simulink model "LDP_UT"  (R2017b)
settings: Solver=FixedStepDiscrete  StartTime=0.0  StopTime=10.0  FixedStep=0.01  RelTol=1e-3  EnableMultiTasking=on
undefined symbols (not defined in the file): ASWTYPE_FALSE, ASWTYPE_TRUE, CaCDP_ChrgTempNTCVoltTable_mV, CaCDP_ChrgTempTable_C, CaLDP_InletWtTempTable_C, CaLDP_InletWtVolt_mV, CaLDP_OutletWtTempTable_C, CaLDP_OutletWtVolt_mV, CcLDP_CC2SplyVolt_mV, CcLDP_CC2Uncon2ConTi_ms, CcLDP_CC2VoltThd_mV, CcLDP_DCChrgNegTempHiThrd_C, CcLDP_DCChrgNegTempMaxThrd_mV, CcLDP_DCChrgNegTempMinThrd_mV, CcLDP_DCChrgPosTempHiThrd_C, CcLDP_DCChrgPosTempMaxThrd_mV, CcLDP_DCChrgPosTempMinThrd_mV, CcLDP_DCSplyOnDebTi_ms, CcLDP_DCWakeVolt_V, CcLDP_IntWtTempHiThrd_C, CcLDP_IntWtTempMaxThrd_mV, CcLDP_IntWtTempMinThrd_mV, CcLDP_OutWtTempHiThrd_C, CcLDP_OutWtTempMaxThrd_mV, CcLDP_OutWtTempMinThrd_mV, Enum_CTCCtrCtlConnMode, Enum_LDPCC2St, Enum_LDPChrgGunState, Enum_ODPCCState, LDP_CONST2_NUMB, LDP_RUNTIME_MS
libraries: AIWAYS_Powertrain_BMS_lib x82
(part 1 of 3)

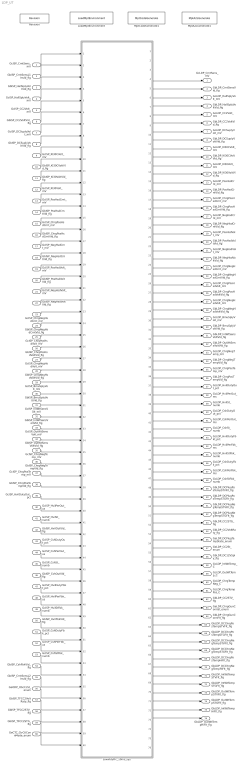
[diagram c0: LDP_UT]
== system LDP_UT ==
  GcISP_CrntSens_mV : Inport
  GbISP_CrntSensL1Invld_flg : Inport  Port=2
  GbISP_HallSplyVoltVld_flg : Inport  Port=3
  GcISP_HallSplyVolt_mV : Inport  Port=4
  GcISP_CC2Volt_mV : Inport  Port=5
  GbISP_CC2VoltVld_flg : Inport  Port=6
  GcISP_DCSuplyVolt_mV : Inport  Port=7
  GbISP_DCSuplyVoltVld_flg : Inport  Port=8
  GcISP_Kl30CVolt_mV : Inport  Port=9
  GbISP_Kl30CVoltVld_flg : Inport  Port=10
  GbISP_Kl30VoltVld_flg : Inport  Port=11
  GcISP_Kl30Volt_mV : Inport  Port=12
  GcISP_PosHsdCrnt_mV : Inport  Port=13
  GbISP_PosHsdCrntVld_flg : Inport  Port=14
  GcISP_ChrgPosHsdCrnt_mV : Inport  Port=15
  GbISP_ChrgPosHsdCrntVld_flg : Inport  Port=16
  GcISP_NegHsdCrnt_mV : Inport  Port=17
  GbISP_NegHsdCrntVld_flg : Inport  Port=18
  GcISP_PosHsdVolt_mV : Inport  Port=19
  GbISP_PosHsdVoltVld_flg : Inport  Port=20
  GcISP_NegHsdVolt_mV : Inport  Port=21
  GbISP_NegHsdVoltVld_flg : Inport  Port=22
  GcISP_ChrgNegHsdCrnt_mV : Inport  Port=23
  GbISP_ChrgNegHsdCrntVld_flg : Inport  Port=24
  GcISP_ChrgPosHsdVolt_mV : Inport  Port=25
  GbISP_ChrgPosHsdVoltVld_flg : Inport  Port=26
  GcISP_ChrgNegHsdVolt_mV : Inport  Port=27
  GbISP_ChrgNegHsdVoltVld_flg : Inport  Port=28
  GcISP_BmuSplyVolt_mV : Inport  Port=29
  GbISP_BmuSplyVoltVld_flg : Inport  Port=30
  GcISP_lntWtSensVolt_mV : Inport  Port=31
  GbISP_lntWtSensVoltVld_flg : Inport  Port=32
  GcISP_OutWtSensVolt_mV : Inport  Port=33
  GbISP_OutWtSensVoltVld_flg : Inport  Port=34
  GcISP_ChrgNegTemp_mV : Inport  Port=35
  GbISP_ChrgNegTempVld_flg : Inport  Port=36
  GcISP_ChrgPosTemp_mV : Inport  Port=37
  GbISP_ChrgPosTempVld_flg : Inport  Port=38
  GcISP_HvilDutyOut_pct : Inport  Port=39
  GcISP_HvilPerOut_us : Inport  Port=40
  GcISP_HvilSt_numb : Inport  Port=41
  GbISP_HvilOutVld_flg : Inport  Port=42
  GcISP_CshDutyOut_pct : Inport  Port=43
  GcISP_CshPerOut_us : Inport  Port=44
  GcISP_CshSt_numb : Inport  Port=45
  GbISP_CshOutVld_flg : Inport  Port=46
  GcISP_HvilDutyFbkt_pct : Inport  Port=47
  GcISP_HvilPerFbk_us : Inport  Port=48
  GcISP_HvilStFbk_numb : Inport  Port=49
  GbISP_HvilFbkVld_flg : Inport  Port=50
  GcISP_CshDutyFbk_pct : Inport  Port=51
  GcISP_CshPerFbk_us : Inport  Port=52
  GcISP_CshStFbk_numb : Inport  Port=53
  GbISP_CshFbkVld_flg : Inport  Port=54
  GbISP_CrntSensL2Invld_flg : Inport  Port=55
  GeODP_ObcCcSt_enum : Inport  Port=56
  GbISP_TFCC2VoltRaty_flg : Inport  Port=57
  GbISP_TFCC2STV_flg : Inport  Port=58
  GbISP_TFCC2STG_flg : Inport  Port=59
  GeCTC_CtrCtlConnMode_enum : Inport  Port=60
  LoadMptEnvironment : AIWAYS_Powertrain_BMS_lib/Config/LoadMptEnvironment  ProjectName=Comm  SuppierID=NewPlatformUAES
  LowVolyPrc_10ms_sys : Subsystem
  MptA2LGenerate1 : AIWAYS_Powertrain_BMS_lib/Config/MptA2LGenerate  SystemSampleTime=-1
  MptCodeGenerate1 : AIWAYS_Powertrain_BMS_lib/Config/MptCodeGenerate  SystemSampleTime=-1
  Revision : AIWAYS_Powertrain_BMS_lib/Config/Revision  curVersion='M104C110'  newVersion='M104C110'
  GcLDP_CrntSens_mV : Outport
  GbLDP_CrntSensVld_flg : Outport  Port=2
  GcLDP_HallSplyVolt_mV : Outport  Port=3
  GbLDP_HallSplyVoltVld_flg : Outport  Port=4
  GcLDP_CC2Volt_mV : Outport  Port=5
  GbLDP_CC2VoltVld_flg : Outport  Port=6
  GcLDP_DCSuplyVolt_mV : Outport  Port=7
  GbLDP_DCSuplyVoltVld_flg : Outport  Port=8
  GcLDP_Kl30CVolt_mV : Outport  Port=9
  GbLDP_Kl30CVoltVld_flg : Outport  Port=10
  GcLDP_Kl30Volt_mV : Outport  Port=11
  GbLDP_Kl30VoltVld_flg : Outport  Port=12
  GcLDP_PosHsdCrnt_mV : Outport  Port=13
  GbLDP_PosHsdCrntVld_flg : Outport  Port=14
  GcLDP_ChrgPosHsdCrnt_mV : Outport  Port=15
  GbLDP_ChrgPosHsdCrntVld_flg : Outport  Port=16
  GcLDP_NegHsdCrnt_mV : Outport  Port=17
  GbLDP_NegHsdCrntVld_flg : Outport  Port=18
  GcLDP_PosHsdVolt_mV : Outport  Port=19
  GbLDP_PosHsdVoltVld_flg : Outport  Port=20
  GcLDP_NegHsdVolt_mV : Outport  Port=21
  GbLDP_NegHsdVoltVld_flg : Outport  Port=22
  GcLDP_ChrgNegHsdCrnt_mV : Outport  Port=23
  GbLDP_ChrgNegHsdCrntVld_flg : Outport  Port=24
  GcLDP_ChrgPosHsdVolt_mV : Outport  Port=25
  GbLDP_ChrgPosHsdVoltVld_flg : Outport  Port=26
  GcLDP_ChrgNegHsdVolt_mV : Outport  Port=27
  GbLDP_ChrgNegHsdVoltVld_flg : Outport  Port=28
  GcLDP_BmuSplyVolt_mV : Outport  Port=29
  GbLDP_BmuSplyVoltVld_flg : Outport  Port=30
  GbLDP_lntWtSensVoltVld_flg : Outport  Port=31
  GbLDP_OutWtSensVoltVld_flg : Outport  Port=32
  GcLDP_ChrgNegTemp_mV : Outport  Port=33
  GbLDP_ChrgNegTempVld_flg : Outport  Port=34
  GcLDP_ChrgPosTemp_mV : Outport  Port=35
  GbLDP_ChrgPosTempVld_flg : Outport  Port=36
  GcLDP_HvilDutyOut_pct : Outport  Port=37
  GcLDP_HvilPerOut_ms : Outport  Port=38
  GcLDP_HvilSt_numb : Outport  Port=39
  GcLDP_CshDutyOut_pct : Outport  Port=40
  GcLDP_CshPerOut_ms : Outport  Port=41
  GcLDP_CshSt_numb : Outport  Port=42
  GcLDP_HvilDutyFbkt_pct : Outport  Port=43
  GcLDP_HvilPerFbk_ms : Outport  Port=44
  GcLDP_HvilStFbk_numb : Outport  Port=45
  GcLDP_CshDutyFbk_pct : Outport  Port=46
  GcLDP_CshPerFbk_ms : Outport  Port=47
  GcLDP_CshStFbk_numb : Outport  Port=48
  GbLDP_DCPlugPosTempSTVFlt_flg : Outport  Port=49
  GbLDP_DCPlugPosTempSTGFlt_flg : Outport  Port=50
  GbLDP_DCPlugNegTempSTVFlt_flg : Outport  Port=51
  GbLDP_DCPlugNegTempSTGFlt_flg : Outport  Port=52
  GbLDP_CC2STG_flg : Outport  Port=53
  GbLDP_CC2VoltRaty_flg : Outport  Port=54
  GeLDP_DCPlugTempState_enum : Outport  Port=55
  GbLDP_DC12VSply_flg : Outport  Port=56
  GeLDP_CC2St_enum : Outport  Port=57
  GcLDP_lntWtTemp_C : Outport  Port=58
  GcLDP_OutWtTemp_C : Outport  Port=59
  GcLDP_ChrgTempNeg_C : Outport  Port=60
  GcLDP_ChrgTempPos_C : Outport  Port=61
  GbLDP_CC2STV_flg : Outport  Port=62
  GeLDP_ChrgGunConnSt_enum : Outport  Port=63
  GbLDP_ChrgGunConnFlt_flg : Outport  Port=64
  GbLDP_DCChrgPosTempSTVFlt_flg : Outport  Port=65
  GbLDP_DCChrgPosTempSTGFlt_flg : Outport  Port=66
  GbLDP_DCChrgNegTempSTVFlt_flg : Outport  Port=67
  GbLDP_DCChrgNegTempSTGFlt_flg : Outport  Port=68
  GbLDP_DCChrgPosTempHiFlt_flg : Outport  Port=69
  GbLDP_DCChrgNegTempHiFlt_flg : Outport  Port=70
  GbLDP_IntWtTempSTVFlt_flg : Outport  Port=71
  GbLDP_IntWtTempSTGFlt_flg : Outport  Port=72
  GbLDP_OutWtTempSTVFlt_flg : Outport  Port=73
  GbLDP_OutWtTempSTGFlt_flg : Outport  Port=74
  GbLDP_IntWtTempHiFlt_flg : Outport  Port=75
  GbLDP_OutWtTempHiFlt_flg : Outport  Port=76
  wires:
  GbISP_DCSuplyVoltVld_flg/1 -> LowVolyPrc_10ms_sys/8(GbISP_DCSuplyVoltVld_flg)
  GbISP_CC2VoltVld_flg/1 -> LowVolyPrc_10ms_sys/6(GbISP_CC2VoltVld_flg)
  LowVolyPrc_10ms_sys/47(GcLDP_CshPerFbk_ms) -> GcLDP_CshPerFbk_ms/1
  LowVolyPrc_10ms_sys/66(GbLDP_DCChrgPosTempSTGFlt_flg) -> GbLDP_DCChrgPosTempSTGFlt_flg/1
  LowVolyPrc_10ms_sys/19(GcLDP_PosHsdVolt_mV) -> GcLDP_PosHsdVolt_mV/1
  GbISP_TFCC2VoltRaty_flg/1 -> LowVolyPrc_10ms_sys/57(GbISP_TFCC2VoltRaty_flg)
  GbISP_PosHsdVoltVld_flg/1 -> LowVolyPrc_10ms_sys/20(GbISP_PosHsdVoltVld_flg)
  LowVolyPrc_10ms_sys/1(GcLDP_CrntSens_mV) -> GcLDP_CrntSens_mV/1
  GcISP_ChrgNegHsdCrnt_mV/1 -> LowVolyPrc_10ms_sys/23(GcISP_ChrgNegHsdCrnt_mV)
  LowVolyPrc_10ms_sys/44(GcLDP_HvilPerFbk_ms) -> GcLDP_HvilPerFbk_ms/1
  LowVolyPrc_10ms_sys/12(GbLDP_Kl30VoltVld_flg) -> GbLDP_Kl30VoltVld_flg/1
  LowVolyPrc_10ms_sys/3(GcLDP_HallSplyVolt_mV) -> GcLDP_HallSplyVolt_mV/1
  LowVolyPrc_10ms_sys/5(GcLDP_CC2Volt_mV) -> GcLDP_CC2Volt_mV/1
  GeCTC_CtrCtlConnMode_enum/1 -> LowVolyPrc_10ms_sys/60(GeCTC_CtrCtlConnMode_enum)
  GcISP_NegHsdVolt_mV/1 -> LowVolyPrc_10ms_sys/21(GcISP_NegHsdVolt_mV)
  LowVolyPrc_10ms_sys/56(GeLDP_CC2St_enum) -> GeLDP_CC2St_enum/1
  GbISP_NegHsdVoltVld_flg/1 -> LowVolyPrc_10ms_sys/22(GbISP_NegHsdVoltVld_flg)
  GcISP_BmuSplyVolt_mV/1 -> LowVolyPrc_10ms_sys/29(GcISP_BmuSplyVolt_mV)
  LowVolyPrc_10ms_sys/36(GbLDP_ChrgPosTempVld_flg) -> GbLDP_ChrgPosTempVld_flg/1
  LowVolyPrc_10ms_sys/24(GbLDP_ChrgNegHsdCrntVld_flg) -> GbLDP_ChrgNegHsdCrntVld_flg/1
  GcISP_NegHsdCrnt_mV/1 -> LowVolyPrc_10ms_sys/17(GcISP_NegHsdCrnt_mV)
  GbISP_TFCC2STG_flg/1 -> LowVolyPrc_10ms_sys/59(GbISP_TFCC2STG_flg)
  LowVolyPrc_10ms_sys/15(GcLDP_ChrgPosHsdCrnt_mV) -> GcLDP_ChrgPosHsdCrnt_mV/1
  LowVolyPrc_10ms_sys/51(GbLDP_DCPlugNegTempSTVFlt_flg) -> GbLDP_DCPlugNegTempSTVFlt_flg/1
  LowVolyPrc_10ms_sys/45(GcLDP_HvilStFbk_numb) -> GcLDP_HvilStFbk_numb/1
  LowVolyPrc_10ms_sys/11(GcLDP_Kl30Volt_mV) -> GcLDP_Kl30Volt_mV/1
  LowVolyPrc_10ms_sys/37(GcLDP_HvilDutyOut_pct) -> GcLDP_HvilDutyOut_pct/1
  GbISP_BmuSplyVoltVld_flg/1 -> LowVolyPrc_10ms_sys/30(GbISP_BmuSplyVoltVld_flg)
  LowVolyPrc_10ms_sys/65(GbLDP_DCChrgPosTempSTVFlt_flg) -> GbLDP_DCChrgPosTempSTVFlt_flg/1
  GbISP_HallSplyVoltVld_flg/1 -> LowVolyPrc_10ms_sys/3(GbISP_HallSplyVoltVld_flg)
  LowVolyPrc_10ms_sys/63(GeLDP_ChrgGunConnSt_enum) -> GeLDP_ChrgGunConnSt_enum/1
  GeODP_ObcCcSt_enum/1 -> LowVolyPrc_10ms_sys/56(GeODP_ObcCcSt_enum)
  GbISP_CshOutVld_flg/1 -> LowVolyPrc_10ms_sys/46(GbISP_CshOutVld_flg)
  LowVolyPrc_10ms_sys/34(GbLDP_ChrgNegTempVld_flg) -> GbLDP_ChrgNegTempVld_flg/1
  GbISP_CrntSensL1Invld_flg/1 -> LowVolyPrc_10ms_sys/2(GbISP_CrntSensL1Invld_flg)
  LowVolyPrc_10ms_sys/25(GcLDP_ChrgPosHsdVolt_mV) -> GcLDP_ChrgPosHsdVolt_mV/1
  LowVolyPrc_10ms_sys/22(GbLDP_NegHsdVoltVld_flg) -> GbLDP_NegHsdVoltVld_flg/1
  LowVolyPrc_10ms_sys/16(GbLDP_ChrgPosHsdCrntVld_flg) -> GbLDP_ChrgPosHsdCrntVld_flg/1
  GcISP_PosHsdCrnt_mV/1 -> LowVolyPrc_10ms_sys/13(GcISP_PosHsdCrnt_mV)
  LowVolyPrc_10ms_sys/20(GbLDP_PosHsdVoltVld_flg) -> GbLDP_PosHsdVoltVld_flg/1
  GcISP_DCSuplyVolt_mV/1 -> LowVolyPrc_10ms_sys/7(GcISP_DCSuplyVolt_mV)
  LowVolyPrc_10ms_sys/18(GbLDP_NegHsdCrntVld_flg) -> GbLDP_NegHsdCrntVld_flg/1
  LowVolyPrc_10ms_sys/14(GbLDP_PosHsdCrntVld_flg) -> GbLDP_PosHsdCrntVld_flg/1
  LowVolyPrc_10ms_sys/21(GcLDP_NegHsdVolt_mV) -> GcLDP_NegHsdVolt_mV/1
  GbISP_PosHsdCrntVld_flg/1 -> LowVolyPrc_10ms_sys/14(GbISP_PosHsdCrntVld_flg)
  LowVolyPrc_10ms_sys/13(GcLDP_PosHsdCrnt_mV) -> GcLDP_PosHsdCrnt_mV/1
  LowVolyPrc_10ms_sys/30(GbLDP_BmuSplyVoltVld_flg) -> GbLDP_BmuSplyVoltVld_flg/1
  LowVolyPrc_10ms_sys/8(GbLDP_DCSuplyVoltVld_flg) -> GbLDP_DCSuplyVoltVld_flg/1
  LowVolyPrc_10ms_sys/54(GbLDP_CC2VoltRaty_flg) -> GbLDP_CC2VoltRaty_flg/1
  LowVolyPrc_10ms_sys/9(GcLDP_Kl30CVolt_mV) -> GcLDP_Kl30CVolt_mV/1
  LowVolyPrc_10ms_sys/26(GbLDP_ChrgPosHsdVoltVld_flg) -> GbLDP_ChrgPosHsdVoltVld_flg/1
  GcISP_Kl30Volt_mV/1 -> LowVolyPrc_10ms_sys/12(GcISP_Kl30Volt_mV)
  GbISP_Kl30VoltVld_flg/1 -> LowVolyPrc_10ms_sys/11(GbISP_Kl30VoltVld_flg)
  GbISP_Kl30CVoltVld_flg/1 -> LowVolyPrc_10ms_sys/10(GbISP_Kl30CVoltVld_flg)
  LowVolyPrc_10ms_sys/17(GcLDP_NegHsdCrnt_mV) -> GcLDP_NegHsdCrnt_mV/1
  GcISP_Kl30CVolt_mV/1 -> LowVolyPrc_10ms_sys/9(GcISP_Kl30CVolt_mV)
  LowVolyPrc_10ms_sys/31(GbLDP_lntWtSensVoltVld_flg) -> GbLDP_lntWtSensVoltVld_flg/1
  LowVolyPrc_10ms_sys/43(GcLDP_HvilDutyFbkt_pct) -> GcLDP_HvilDutyFbkt_pct/1
  LowVolyPrc_10ms_sys/7(GcLDP_DCSuplyVolt_mV) -> GcLDP_DCSuplyVolt_mV/1
  LowVolyPrc_10ms_sys/35(GcLDP_ChrgPosTemp_mV) -> GcLDP_ChrgPosTemp_mV/1
  LowVolyPrc_10ms_sys/32(GbLDP_OutWtSensVoltVld_flg) -> GbLDP_OutWtSensVoltVld_flg/1
  GbISP_ChrgPosHsdCrntVld_flg/1 -> LowVolyPrc_10ms_sys/16(GbISP_ChrgPosHsdCrntVld_flg)
  LowVolyPrc_10ms_sys/28(GbLDP_ChrgNegHsdVoltVld_flg) -> GbLDP_ChrgNegHsdVoltVld_flg/1
  GbISP_ChrgNegHsdCrntVld_flg/1 -> LowVolyPrc_10ms_sys/24(GbISP_ChrgNegHsdCrntVld_flg)
  GcISP_PosHsdVolt_mV/1 -> LowVolyPrc_10ms_sys/19(GcISP_PosHsdVolt_mV)
  LowVolyPrc_10ms_sys/10(GbLDP_Kl30CVoltVld_flg) -> GbLDP_Kl30CVoltVld_flg/1
  GcISP_CshPerFbk_us/1 -> LowVolyPrc_10ms_sys/52(GcISP_CshPerFbk_us)
  GbISP_HvilFbkVld_flg/1 -> LowVolyPrc_10ms_sys/50(GbISP_HvilFbkVld_flg)
  LowVolyPrc_10ms_sys/70(GbLDP_DCChrgNegTempHiFlt_flg) -> GbLDP_DCChrgNegTempHiFlt_flg/1
  GcISP_HvilPerOut_us/1 -> LowVolyPrc_10ms_sys/40(GcISP_HvilPerOut_us)
  GcISP_CshDutyOut_pct/1 -> LowVolyPrc_10ms_sys/43(GcISP_CshDutyOut_pct)
  LowVolyPrc_10ms_sys/49(GbLDP_DCPlugPosTempSTVFlt_flg) -> GbLDP_DCPlugPosTempSTVFlt_flg/1
  LowVolyPrc_10ms_sys/57(GbLDP_DC12VSply_flg) -> GbLDP_DC12VSply_flg/1
  GcISP_OutWtSensVolt_mV/1 -> LowVolyPrc_10ms_sys/33(GcISP_OutWtSensVolt_mV)
  LowVolyPrc_10ms_sys/40(GcLDP_CshDutyOut_pct) -> GcLDP_CshDutyOut_pct/1
  GbISP_ChrgNegTempVld_flg/1 -> LowVolyPrc_10ms_sys/36(GbISP_ChrgNegTempVld_flg)
  GcISP_ChrgPosHsdCrnt_mV/1 -> LowVolyPrc_10ms_sys/15(GcISP_ChrgPosHsdCrnt_mV)
  LowVolyPrc_10ms_sys/61(GcLDP_ChrgTempPos_C) -> GcLDP_ChrgTempPos_C/1
  GcISP_HvilDutyFbkt_pct/1 -> LowVolyPrc_10ms_sys/47(GcISP_HvilDutyFbkt_pct)
  LowVolyPrc_10ms_sys/52(GbLDP_DCPlugNegTempSTGFlt_flg) -> GbLDP_DCPlugNegTempSTGFlt_flg/1
  GcISP_ChrgPosTemp_mV/1 -> LowVolyPrc_10ms_sys/37(GcISP_ChrgPosTemp_mV)
  LowVolyPrc_10ms_sys/60(GcLDP_ChrgTempNeg_C) -> GcLDP_ChrgTempNeg_C/1
  LowVolyPrc_10ms_sys/41(GcLDP_CshPerOut_ms) -> GcLDP_CshPerOut_ms/1
  GbISP_CrntSensL2Invld_flg/1 -> LowVolyPrc_10ms_sys/55(GbISP_CrntSensL2Invld_flg)
  LowVolyPrc_10ms_sys/48(GcLDP_CshStFbk_numb) -> GcLDP_CshStFbk_numb/1
  LowVolyPrc_10ms_sys/2(GbLDP_CrntSensVld_flg) -> GbLDP_CrntSensVld_flg/1
  LowVolyPrc_10ms_sys/74(GbLDP_OutWtTempSTGFlt_flg) -> GbLDP_OutWtTempSTGFlt_flg/1
  GcISP_ChrgNegTemp_mV/1 -> LowVolyPrc_10ms_sys/35(GcISP_ChrgNegTemp_mV)
  LowVolyPrc_10ms_sys/59(GcLDP_OutWtTemp_C) -> GcLDP_OutWtTemp_C/1
  LowVolyPrc_10ms_sys/42(GcLDP_CshSt_numb) -> GcLDP_CshSt_numb/1
  LowVolyPrc_10ms_sys/76(GbLDP_OutWtTempHiFlt_flg) -> GbLDP_OutWtTempHiFlt_flg/1
  GcISP_ChrgNegHsdVolt_mV/1 -> LowVolyPrc_10ms_sys/27(GcISP_ChrgNegHsdVolt_mV)
  GcISP_HallSplyVolt_mV/1 -> LowVolyPrc_10ms_sys/4(GcISP_HallSplyVolt_mV)
  LowVolyPrc_10ms_sys/71(GbLDP_IntWtTempSTVFlt_flg) -> GbLDP_IntWtTempSTVFlt_flg/1
  LowVolyPrc_10ms_sys/75(GbLDP_IntWtTempHiFlt_flg) -> GbLDP_IntWtTempHiFlt_flg/1
  GbISP_OutWtSensVoltVld_flg/1 -> LowVolyPrc_10ms_sys/34(GbISP_OutWtSensVoltVld_flg)
  GcISP_HvilStFbk_numb/1 -> LowVolyPrc_10ms_sys/49(GcISP_HvilStFbk_numb)
  LowVolyPrc_10ms_sys/67(GbLDP_DCChrgNegTempSTVFlt_flg) -> GbLDP_DCChrgNegTempSTVFlt_flg/1
  GbISP_ChrgPosHsdVoltVld_flg/1 -> LowVolyPrc_10ms_sys/26(GbISP_ChrgPosHsdVoltVld_flg)
  LowVolyPrc_10ms_sys/33(GcLDP_ChrgNegTemp_mV) -> GcLDP_ChrgNegTemp_mV/1
  GbISP_TFCC2STV_flg/1 -> LowVolyPrc_10ms_sys/58(GbISP_TFCC2STV_flg)
  GcISP_CshSt_numb/1 -> LowVolyPrc_10ms_sys/45(GcISP_CshSt_numb)
  GcISP_HvilPerFbk_us/1 -> LowVolyPrc_10ms_sys/48(GcISP_HvilPerFbk_us)
  LowVolyPrc_10ms_sys/53(GbLDP_CC2STG_flg) -> GbLDP_CC2STG_flg/1
  GbISP_lntWtSensVoltVld_flg/1 -> LowVolyPrc_10ms_sys/32(GbISP_lntWtSensVoltVld_flg)
  LowVolyPrc_10ms_sys/73(GbLDP_OutWtTempSTVFlt_flg) -> GbLDP_OutWtTempSTVFlt_flg/1
  LowVolyPrc_10ms_sys/39(GcLDP_HvilSt_numb) -> GcLDP_HvilSt_numb/1
  LowVolyPrc_10ms_sys/64(GbLDP_ChrgGunConnFlt_flg) -> GbLDP_ChrgGunConnFlt_flg/1
  GbISP_NegHsdCrntVld_flg/1 -> LowVolyPrc_10ms_sys/18(GbISP_NegHsdCrntVld_flg)
  GcISP_HvilSt_numb/1 -> LowVolyPrc_10ms_sys/41(GcISP_HvilSt_numb)
  GcISP_ChrgPosHsdVolt_mV/1 -> LowVolyPrc_10ms_sys/25(GcISP_ChrgPosHsdVolt_mV)
  GcISP_CshDutyFbk_pct/1 -> LowVolyPrc_10ms_sys/51(GcISP_CshDutyFbk_pct)
  LowVolyPrc_10ms_sys/55(GeLDP_DCPlugTempState_enum) -> GeLDP_DCPlugTempState_enum/1
  LowVolyPrc_10ms_sys/38(GcLDP_HvilPerOut_ms) -> GcLDP_HvilPerOut_ms/1
  GcISP_lntWtSensVolt_mV/1 -> LowVolyPrc_10ms_sys/31(GcISP_lntWtSensVolt_mV)
  GbISP_HvilOutVld_flg/1 -> LowVolyPrc_10ms_sys/42(GbISP_HvilOutVld_flg)
  LowVolyPrc_10ms_sys/72(GbLDP_IntWtTempSTGFlt_flg) -> GbLDP_IntWtTempSTGFlt_flg/1
  GbISP_CshFbkVld_flg/1 -> LowVolyPrc_10ms_sys/54(GbISP_CshFbkVld_flg)
  GcISP_CC2Volt_mV/1 -> LowVolyPrc_10ms_sys/5(GcISP_CC2Volt_mV)
  LowVolyPrc_10ms_sys/58(GcLDP_lntWtTemp_C) -> GcLDP_lntWtTemp_C/1
  LowVolyPrc_10ms_sys/29(GcLDP_BmuSplyVolt_mV) -> GcLDP_BmuSplyVolt_mV/1
  LowVolyPrc_10ms_sys/6(GbLDP_CC2VoltVld_flg) -> GbLDP_CC2VoltVld_flg/1
  LowVolyPrc_10ms_sys/50(GbLDP_DCPlugPosTempSTGFlt_flg) -> GbLDP_DCPlugPosTempSTGFlt_flg/1
  GcISP_CshPerOut_us/1 -> LowVolyPrc_10ms_sys/44(GcISP_CshPerOut_us)
  LowVolyPrc_10ms_sys/4(GbLDP_HallSplyVoltVld_flg) -> GbLDP_HallSplyVoltVld_flg/1
  LowVolyPrc_10ms_sys/27(GcLDP_ChrgNegHsdVolt_mV) -> GcLDP_ChrgNegHsdVolt_mV/1
  GcISP_CshStFbk_numb/1 -> LowVolyPrc_10ms_sys/53(GcISP_CshStFbk_numb)
  LowVolyPrc_10ms_sys/68(GbLDP_DCChrgNegTempSTGFlt_flg) -> GbLDP_DCChrgNegTempSTGFlt_flg/1
  GbISP_ChrgPosTempVld_flg/1 -> LowVolyPrc_10ms_sys/38(GbISP_ChrgPosTempVld_flg)
  GcISP_CrntSens_mV/1 -> LowVolyPrc_10ms_sys/1(GcISP_CrntSens_mV)
  LowVolyPrc_10ms_sys/69(GbLDP_DCChrgPosTempHiFlt_flg) -> GbLDP_DCChrgPosTempHiFlt_flg/1
  GbISP_ChrgNegHsdVoltVld_flg/1 -> LowVolyPrc_10ms_sys/28(GbISP_ChrgNegHsdVoltVld_flg)
  GcISP_HvilDutyOut_pct/1 -> LowVolyPrc_10ms_sys/39(GcISP_HvilDutyOut_pct)
  LowVolyPrc_10ms_sys/46(GcLDP_CshDutyFbk_pct) -> GcLDP_CshDutyFbk_pct/1
  LowVolyPrc_10ms_sys/62(GbLDP_CC2STV_flg) -> GbLDP_CC2STV_flg/1
  LowVolyPrc_10ms_sys/23(GcLDP_ChrgNegHsdCrnt_mV) -> GcLDP_ChrgNegHsdCrnt_mV/1

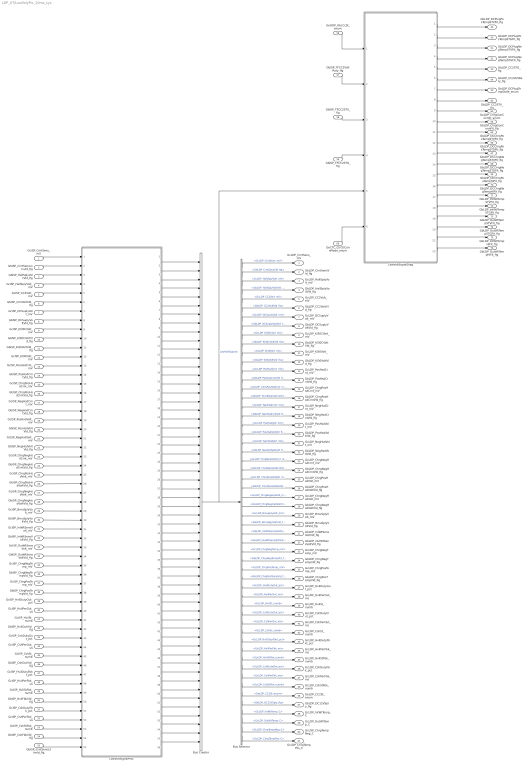
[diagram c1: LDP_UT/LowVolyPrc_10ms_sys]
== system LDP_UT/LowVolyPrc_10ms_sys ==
  GcISP_CrntSens_mV : Inport
  GbISP_CrntSensL1Invld_flg : Inport  Port=2
  GbISP_HallSplyVoltVld_flg : Inport  Port=3
  GcISP_HallSplyVolt_mV : Inport  Port=4
  GcISP_CC2Volt_mV : Inport  Port=5
  GbISP_CC2VoltVld_flg : Inport  Port=6
  GcISP_DCSuplyVolt_mV : Inport  Port=7
  GbISP_DCSuplyVoltVld_flg : Inport  Port=8
  GcISP_Kl30CVolt_mV : Inport  Port=9
  GbISP_Kl30CVoltVld_flg : Inport  Port=10
  GbISP_Kl30VoltVld_flg : Inport  Port=11
  GcISP_Kl30Volt_mV : Inport  Port=12
  GcISP_PosHsdCrnt_mV : Inport  Port=13
  GbISP_PosHsdCrntVld_flg : Inport  Port=14
  GcISP_ChrgPosHsdCrnt_mV : Inport  Port=15
  GbISP_ChrgPosHsdCrntVld_flg : Inport  Port=16
  GcISP_NegHsdCrnt_mV : Inport  Port=17
  GbISP_NegHsdCrntVld_flg : Inport  Port=18
  GcISP_PosHsdVolt_mV : Inport  Port=19
  GbISP_PosHsdVoltVld_flg : Inport  Port=20
  GcISP_NegHsdVolt_mV : Inport  Port=21
  GbISP_NegHsdVoltVld_flg : Inport  Port=22
  GcISP_ChrgNegHsdCrnt_mV : Inport  Port=23
  GbISP_ChrgNegHsdCrntVld_flg : Inport  Port=24
  GcISP_ChrgPosHsdVolt_mV : Inport  Port=25
  GbISP_ChrgPosHsdVoltVld_flg : Inport  Port=26
  GcISP_ChrgNegHsdVolt_mV : Inport  Port=27
  GbISP_ChrgNegHsdVoltVld_flg : Inport  Port=28
  GcISP_BmuSplyVolt_mV : Inport  Port=29
  GbISP_BmuSplyVoltVld_flg : Inport  Port=30
  GcISP_lntWtSensVolt_mV : Inport  Port=31
  GbISP_lntWtSensVoltVld_flg : Inport  Port=32
  GcISP_OutWtSensVolt_mV : Inport  Port=33
  GbISP_OutWtSensVoltVld_flg : Inport  Port=34
  GcISP_ChrgNegTemp_mV : Inport  Port=35
  GbISP_ChrgNegTempVld_flg : Inport  Port=36
  GcISP_ChrgPosTemp_mV : Inport  Port=37
  GbISP_ChrgPosTempVld_flg : Inport  Port=38
  GcISP_HvilDutyOut_pct : Inport  Port=39
  GcISP_HvilPerOut_us : Inport  Port=40
  GcISP_HvilSt_numb : Inport  Port=41
  GbISP_HvilOutVld_flg : Inport  Port=42
  GcISP_CshDutyOut_pct : Inport  Port=43
  GcISP_CshPerOut_us : Inport  Port=44
  GcISP_CshSt_numb : Inport  Port=45
  GbISP_CshOutVld_flg : Inport  Port=46
  GcISP_HvilDutyFbkt_pct : Inport  Port=47
  GcISP_HvilPerFbk_us : Inport  Port=48
  GcISP_HvilStFbk_numb : Inport  Port=49
  GbISP_HvilFbkVld_flg : Inport  Port=50
  GcISP_CshDutyFbk_pct : Inport  Port=51
  GcISP_CshPerFbk_us : Inport  Port=52
  GcISP_CshStFbk_numb : Inport  Port=53
  GbISP_CshFbkVld_flg : Inport  Port=54
  GbISP_CrntSensL2Invld_flg : Inport  Port=55
  GeODP_ObcCcSt_enum : Inport  Port=56
  GbISP_TFCC2VoltRaty_flg : Inport  Port=57
  GbISP_TFCC2STV_flg : Inport  Port=58
  GbISP_TFCC2STG_flg : Inport  Port=59
  GeCTC_CtrCtlConnMode_enum : Inport  Port=60
  Bus Creator : BusCreator  Inputs=56
  Bus Selector : BusSelector  OutputSignals=GcLDP_CrntSens_mV,GbLDP_CrntSensVld_flg,GcLDP_HallSplyVolt_mV,GbLDP_HallSplyVoltVld_flg,GcLDP_CC2Volt_mV,GbLDP_CC2VoltVld_flg,GcLDP_DCSuplyVolt_mV,GbLDP_DCSuplyVoltVld_flg,GcLDP_Kl30CVolt_mV,GbLDP_Kl30CVoltVld_flg,GcLDP_Kl30Volt_mV,GbLDP_Kl30VoltVld_flg,GcLDP_PosHsdCrnt_mV,GbLDP_PosHsdCrntVld_flg,GcLDP_ChrgPosHsdCrnt_mV,GbLDP_ChrgPosHsdCrntVld_flg,GcLDP_NegHsdCrnt_mV,GbLDP_NegHsdCrntVld_flg,GcLDP_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
  LowVoltSignalDiag : Subsystem
  LowVoltSignalProc : Subsystem
  GcLDP_CrntSens_mV : Outport
  GbLDP_CrntSensVld_flg : Outport  Port=2
  GcLDP_HallSplyVolt_mV : Outport  Port=3
  GbLDP_HallSplyVoltVld_flg : Outport  Port=4
  GcLDP_CC2Volt_mV : Outport  Port=5
  GbLDP_CC2VoltVld_flg : Outport  Port=6
  GcLDP_DCSuplyVolt_mV : Outport  Port=7
  GbLDP_DCSuplyVoltVld_flg : Outport  Port=8
  GcLDP_Kl30CVolt_mV : Outport  Port=9
  GbLDP_Kl30CVoltVld_flg : Outport  Port=10
  GcLDP_Kl30Volt_mV : Outport  Port=11
  GbLDP_Kl30VoltVld_flg : Outport  Port=12
  GcLDP_PosHsdCrnt_mV : Outport  Port=13
  GbLDP_PosHsdCrntVld_flg : Outport  Port=14
  GcLDP_ChrgPosHsdCrnt_mV : Outport  Port=15
  GbLDP_ChrgPosHsdCrntVld_flg : Outport  Port=16
  GcLDP_NegHsdCrnt_mV : Outport  Port=17
  GbLDP_NegHsdCrntVld_flg : Outport  Port=18
  GcLDP_PosHsdVolt_mV : Outport  Port=19
  GbLDP_PosHsdVoltVld_flg : Outport  Port=20
  GcLDP_NegHsdVolt_mV : Outport  Port=21
  GbLDP_NegHsdVoltVld_flg : Outport  Port=22
  GcLDP_ChrgNegHsdCrnt_mV : Outport  Port=23
  GbLDP_ChrgNegHsdCrntVld_flg : Outport  Port=24
  GcLDP_ChrgPosHsdVolt_mV : Outport  Port=25
  GbLDP_ChrgPosHsdVoltVld_flg : Outport  Port=26
  GcLDP_ChrgNegHsdVolt_mV : Outport  Port=27
  GbLDP_ChrgNegHsdVoltVld_flg : Outport  Port=28
  GcLDP_BmuSplyVolt_mV : Outport  Port=29
  GbLDP_BmuSplyVoltVld_flg : Outport  Port=30
  GbLDP_lntWtSensVoltVld_flg : Outport  Port=31
  GbLDP_OutWtSensVoltVld_flg : Outport  Port=32
  GcLDP_ChrgNegTemp_mV : Outport  Port=33
  GbLDP_ChrgNegTempVld_flg : Outport  Port=34
  GcLDP_ChrgPosTemp_mV : Outport  Port=35
  GbLDP_ChrgPosTempVld_flg : Outport  Port=36
  GcLDP_HvilDutyOut_pct : Outport  Port=37
  GcLDP_HvilPerOut_ms : Outport  Port=38
  GcLDP_HvilSt_numb : Outport  Port=39
  GcLDP_CshDutyOut_pct : Outport  Port=40
  GcLDP_CshPerOut_ms : Outport  Port=41
  GcLDP_CshSt_numb : Outport  Port=42
  GcLDP_HvilDutyFbkt_pct : Outport  Port=43
  GcLDP_HvilPerFbk_ms : Outport  Port=44
  GcLDP_HvilStFbk_numb : Outport  Port=45
  GcLDP_CshDutyFbk_pct : Outport  Port=46
  GcLDP_CshPerFbk_ms : Outport  Port=47
  GcLDP_CshStFbk_numb : Outport  Port=48
  GbLDP_DCPlugPosTempSTVFlt_flg : Outport  Port=49
  GbLDP_DCPlugPosTempSTGFlt_flg : Outport  Port=50
  GbLDP_DCPlugNegTempSTVFlt_flg : Outport  Port=51
  GbLDP_DCPlugNegTempSTGFlt_flg : Outport  Port=52
  GbLDP_CC2STG_flg : Outport  Port=53
  GbLDP_CC2VoltRaty_flg : Outport  Port=54
  GeLDP_DCPlugTempState_enum : Outport  Port=55
  GeLDP_CC2St_enum : Outport  Port=56
  GbLDP_DC12VSply_flg : Outport  Port=57
  GcLDP_lntWtTemp_C : Outport  Port=58
  GcLDP_OutWtTemp_C : Outport  Port=59
  GcLDP_ChrgTempNeg_C : Outport  Port=60
  GcLDP_ChrgTempPos_C : Outport  Port=61
  GbLDP_CC2STV_flg : Outport  Port=62
  GeLDP_ChrgGunConnSt_enum : Outport  Port=63
  GbLDP_ChrgGunConnFlt_flg : Outport  Port=64
  GbLDP_DCChrgPosTempSTVFlt_flg : Outport  Port=65
  GbLDP_DCChrgPosTempSTGFlt_flg : Outport  Port=66
  GbLDP_DCChrgNegTempSTVFlt_flg : Outport  Port=67
  GbLDP_DCChrgNegTempSTGFlt_flg : Outport  Port=68
  GbLDP_DCChrgPosTempHiFlt_flg : Outport  Port=69
  GbLDP_DCChrgNegTempHiFlt_flg : Outport  Port=70
  GbLDP_IntWtTempSTVFlt_flg : Outport  Port=71
  GbLDP_IntWtTempSTGFlt_flg : Outport  Port=72
  GbLDP_OutWtTempSTVFlt_flg : Outport  Port=73
  GbLDP_OutWtTempSTGFlt_flg : Outport  Port=74
  GbLDP_IntWtTempHiFlt_flg : Outport  Port=75
  GbLDP_OutWtTempHiFlt_flg : Outport  Port=76
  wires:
  GcISP_CrntSens_mV/1 -> LowVoltSignalProc/1(GcISP_CrntSens_mV)
  GbISP_CrntSensL1Invld_flg/1 -> LowVoltSignalProc/2(GbISP_CrntSensL1Invld_flg)
  GbISP_HallSplyVoltVld_flg/1 -> LowVoltSignalProc/3(GbISP_HallSplyVoltVld_flg)
  GcISP_HallSplyVolt_mV/1 -> LowVoltSignalProc/4(GcISP_HallSplyVolt_mV)
  GcISP_CC2Volt_mV/1 -> LowVoltSignalProc/5(GcISP_CC2Volt_mV)
  GbISP_CC2VoltVld_flg/1 -> LowVoltSignalProc/6(GbISP_CC2VoltVld_flg)
  GcISP_DCSuplyVolt_mV/1 -> LowVoltSignalProc/7(GcISP_DCSuplyVolt_mV)
  GbISP_DCSuplyVoltVld_flg/1 -> LowVoltSignalProc/8(GbISP_DCSuplyVoltVld_flg)
  GbISP_Kl30VoltVld_flg/1 -> LowVoltSignalProc/11(GbISP_Kl30VoltVld_flg)
  GcISP_Kl30Volt_mV/1 -> LowVoltSignalProc/12(GcISP_Kl30Volt_mV)
  GcISP_PosHsdCrnt_mV/1 -> LowVoltSignalProc/13(GcISP_PosHsdCrnt_mV)
  GbISP_PosHsdCrntVld_flg/1 -> LowVoltSignalProc/14(GbISP_PosHsdCrntVld_flg)
  GcISP_ChrgPosHsdCrnt_mV/1 -> LowVoltSignalProc/15(GcISP_ChrgPosHsdCrnt_mV)
  GbISP_ChrgPosHsdCrntVld_flg/1 -> LowVoltSignalProc/16(GbISP_ChrgPosHsdCrntVld_flg)
  GcISP_NegHsdCrnt_mV/1 -> LowVoltSignalProc/17(GcISP_NegHsdCrnt_mV)
  GbISP_NegHsdCrntVld_flg/1 -> LowVoltSignalProc/18(GbISP_NegHsdCrntVld_flg)
  GcISP_PosHsdVolt_mV/1 -> LowVoltSignalProc/19(GcISP_PosHsdVolt_mV)
  GbISP_PosHsdVoltVld_flg/1 -> LowVoltSignalProc/20(GbISP_PosHsdVoltVld_flg)
  GcISP_NegHsdVolt_mV/1 -> LowVoltSignalProc/21(GcISP_NegHsdVolt_mV)
  GbISP_NegHsdVoltVld_flg/1 -> LowVoltSignalProc/22(GbISP_NegHsdVoltVld_flg)
  GcISP_ChrgNegHsdCrnt_mV/1 -> LowVoltSignalProc/23(GcISP_ChrgNegHsdCrnt_mV)
  GbISP_ChrgNegHsdCrntVld_flg/1 -> LowVoltSignalProc/24(GbISP_ChrgNegHsdCrntVld_flg)
  GcISP_ChrgPosHsdVolt_mV/1 -> LowVoltSignalProc/25(GcISP_ChrgPosHsdVolt_mV)
  GbISP_ChrgPosHsdVoltVld_flg/1 -> LowVoltSignalProc/26(GbISP_ChrgPosHsdVoltVld_flg)
  GcISP_ChrgNegHsdVolt_mV/1 -> LowVoltSignalProc/27(GcISP_ChrgNegHsdVolt_mV)
  GbISP_ChrgNegHsdVoltVld_flg/1 -> LowVoltSignalProc/28(GbISP_ChrgNegHsdVoltVld_flg)
  GcISP_BmuSplyVolt_mV/1 -> LowVoltSignalProc/29(GcISP_BmuSplyVolt_mV)
  GbISP_BmuSplyVoltVld_flg/1 -> LowVoltSignalProc/30(GbISP_BmuSplyVoltVld_flg)
  GcISP_lntWtSensVolt_mV/1 -> LowVoltSignalProc/31(GcISP_lntWtSensVolt_mV)
  GbISP_lntWtSensVoltVld_flg/1 -> LowVoltSignalProc/32(GbISP_lntWtSensVoltVld_flg)
  GcISP_OutWtSensVolt_mV/1 -> LowVoltSignalProc/33(GcISP_OutWtSensVolt_mV)
  GbISP_OutWtSensVoltVld_flg/1 -> LowVoltSignalProc/34(GbISP_OutWtSensVoltVld_flg)
  GcISP_ChrgNegTemp_mV/1 -> LowVoltSignalProc/35(GcISP_ChrgNegTemp_mV)
  GbISP_ChrgNegTempVld_flg/1 -> LowVoltSignalProc/36(GbISP_ChrgNegTempVld_flg)
  GcISP_ChrgPosTemp_mV/1 -> LowVoltSignalProc/37(GcISP_ChrgPosTemp_mV)
  GbISP_ChrgPosTempVld_flg/1 -> LowVoltSignalProc/38(GbISP_ChrgPosTempVld_flg)
  GcISP_HvilDutyOut_pct/1 -> LowVoltSignalProc/39(GcISP_HvilDutyOut_pct)
  GcISP_HvilPerOut_us/1 -> LowVoltSignalProc/40(GcISP_HvilPerOut_us)
  GcISP_HvilSt_numb/1 -> LowVoltSignalProc/41(GcISP_HvilSt_numb)
  GcISP_CshDutyOut_pct/1 -> LowVoltSignalProc/43(GcISP_CshDutyOut_pct)
  GcISP_CshPerOut_us/1 -> LowVoltSignalProc/44(GcISP_CshPerOut_us)
  GcISP_CshSt_numb/1 -> LowVoltSignalProc/45(GcISP_CshSt_numb)
  GcISP_HvilDutyFbkt_pct/1 -> LowVoltSignalProc/47(GcISP_HvilDutyFbkt_pct)
  GcISP_HvilPerFbk_us/1 -> LowVoltSignalProc/48(GcISP_HvilPerFbk_us)
  GcISP_HvilStFbk_numb/1 -> LowVoltSignalProc/49(GcISP_HvilStFbk_numb)
  GcISP_CshDutyFbk_pct/1 -> LowVoltSignalProc/51(GcISP_CshDutyFbk_pct)
  GcISP_CshPerFbk_us/1 -> LowVoltSignalProc/52(GcISP_CshPerFbk_us)
  GcISP_CshStFbk_numb/1 -> LowVoltSignalProc/53(GcISP_CshStFbk_numb)
  Bus Creator/1 -> LowVoltSignalDiag/5(LowVoltSignals), Bus Selector/1  "LowVoltSignals"
  Bus Selector/1 -> GcLDP_CrntSens_mV/1  "<GcLDP_CrntSens_mV>"
  Bus Selector/2 -> GbLDP_CrntSensVld_flg/1  "<GbLDP_CrntSensVld_flg>"
  Bus Selector/3 -> GcLDP_HallSplyVolt_mV/1  "<GcLDP_HallSplyVolt_mV>"
  Bus Selector/4 -> GbLDP_HallSplyVoltVld_flg/1  "<GbLDP_HallSplyVoltVld_flg>"
  Bus Selector/5 -> GcLDP_CC2Volt_mV/1  "<GcLDP_CC2Volt_mV>"
  Bus Selector/6 -> GbLDP_CC2VoltVld_flg/1  "<GbLDP_CC2VoltVld_flg>"
  Bus Selector/7 -> GcLDP_DCSuplyVolt_mV/1  "<GcLDP_DCSuplyVolt_mV>"
  Bus Selector/8 -> GbLDP_DCSuplyVoltVld_flg/1  "<GbLDP_DCSuplyVoltVld_flg>"
  Bus Selector/9 -> GcLDP_Kl30CVolt_mV/1  "<GcLDP_Kl30CVolt_mV>"
  Bus Selector/10 -> GbLDP_Kl30CVoltVld_flg/1  "<GbLDP_Kl30CVoltVld_flg>"
  Bus Selector/11 -> GcLDP_Kl30Volt_mV/1  "<GcLDP_Kl30Volt_mV>"
  Bus Selector/12 -> GbLDP_Kl30VoltVld_flg/1  "<GbLDP_Kl30VoltVld_flg>"
  Bus Selector/13 -> GcLDP_PosHsdCrnt_mV/1  "<GcLDP_PosHsdCrnt_mV>"
  Bus Selector/14 -> GbLDP_PosHsdCrntVld_flg/1  "<GbLDP_PosHsdCrntVld_flg>"
  Bus Selector/15 -> GcLDP_ChrgPosHsdCrnt_mV/1  "<GcLDP_ChrgPosHsdCrnt_mV>"
  Bus Selector/16 -> GbLDP_ChrgPosHsdCrntVld_flg/1  "<GbLDP_ChrgPosHsdCrntVld_flg>"
  Bus Selector/17 -> GcLDP_NegHsdCrnt_mV/1  "<GcLDP_NegHsdCrnt_mV>"
  Bus Selector/18 -> GbLDP_NegHsdCrntVld_flg/1  "<GbLDP_NegHsdCrntVld_flg>"
  Bus Selector/19 -> GcLDP_PosHsdVolt_mV/1  "<GcLDP_PosHsdVolt_mV>"
  Bus Selector/20 -> GbLDP_PosHsdVoltVld_flg/1  "<GbLDP_PosHsdVoltVld_flg>"
  Bus Selector/21 -> GcLDP_NegHsdVolt_mV/1  "<GcLDP_NegHsdVolt_mV>"
  Bus Selector/22 -> GbLDP_NegHsdVoltVld_flg/1  "<GbLDP_NegHsdVoltVld_flg>"
  Bus Selector/23 -> GcLDP_ChrgNegHsdCrnt_mV/1  "<GcLDP_ChrgNegHsdCrnt_mV>"
  Bus Selector/24 -> GbLDP_ChrgNegHsdCrntVld_flg/1  "<GbLDP_ChrgNegHsdCrntVld_flg>"
  Bus Selector/25 -> GcLDP_ChrgPosHsdVolt_mV/1  "<GcLDP_ChrgPosHsdVolt_mV>"
  Bus Selector/26 -> GbLDP_ChrgPosHsdVoltVld_flg/1  "<GbLDP_ChrgPosHsdVoltVld_flg>"
  Bus Selector/27 -> GcLDP_ChrgNegHsdVolt_mV/1  "<GcLDP_ChrgNegHsdVolt_mV>"
  Bus Selector/28 -> GbLDP_ChrgNegHsdVoltVld_flg/1  "<GbLDP_ChrgNegHsdVoltVld_flg>"
  Bus Selector/29 -> GcLDP_BmuSplyVolt_mV/1  "<GcLDP_BmuSplyVolt_mV>"
  Bus Selector/30 -> GbLDP_BmuSplyVoltVld_flg/1  "<GbLDP_BmuSplyVoltVld_flg>"
  Bus Selector/31 -> GbLDP_lntWtSensVoltVld_flg/1  "<GbLDP_lntWtSensVoltVld_flg>"
  Bus Selector/32 -> GbLDP_OutWtSensVoltVld_flg/1  "<GbLDP_OutWtSensVoltVld_flg>"
  Bus Selector/33 -> GcLDP_ChrgNegTemp_mV/1  "<GcLDP_ChrgNegTemp_mV>"
  Bus Selector/34 -> GbLDP_ChrgNegTempVld_flg/1  "<GbLDP_ChrgNegTempVld_flg>"
  Bus Selector/35 -> GcLDP_ChrgPosTemp_mV/1  "<GcLDP_ChrgPosTemp_mV>"
  Bus Selector/36 -> GbLDP_ChrgPosTempVld_flg/1  "<GbLDP_ChrgPosTempVld_flg>"
  Bus Selector/37 -> GcLDP_HvilDutyOut_pct/1  "<GcLDP_HvilDutyOut_pct>"
  Bus Selector/38 -> GcLDP_HvilPerOut_ms/1  "<GcLDP_HvilPerOut_ms>"
  Bus Selector/39 -> GcLDP_HvilSt_numb/1  "<GcLDP_HvilSt_numb>"
  Bus Selector/40 -> GcLDP_CshDutyOut_pct/1  "<GcLDP_CshDutyOut_pct>"
  Bus Selector/41 -> GcLDP_CshPerOut_ms/1  "<GcLDP_CshPerOut_ms>"
  Bus Selector/42 -> GcLDP_CshSt_numb/1  "<GcLDP_CshSt_numb>"
  Bus Selector/43 -> GcLDP_HvilDutyFbkt_pct/1  "<GcLDP_HvilDutyFbkt_pct>"
  Bus Selector/44 -> GcLDP_HvilPerFbk_ms/1  "<GcLDP_HvilPerFbk_ms>"
  Bus Selector/45 -> GcLDP_HvilStFbk_numb/1  "<GcLDP_HvilStFbk_numb>"
  Bus Selector/46 -> GcLDP_CshDutyFbk_pct/1  "<GcLDP_CshDutyFbk_pct>"
  Bus Selector/47 -> GcLDP_CshPerFbk_ms/1  "<GcLDP_CshPerFbk_ms>"
  Bus Selector/48 -> GcLDP_CshStFbk_numb/1  "<GcLDP_CshStFbk_numb>"
  LowVoltSignalDiag/1(GbLDP_DCPlugPosTempSTVFlt_flg) -> GbLDP_DCPlugPosTempSTVFlt_flg/1
  LowVoltSignalDiag/2(GbLDP_DCPlugPosTempSTGFlt_flg) -> GbLDP_DCPlugPosTempSTGFlt_flg/1
  LowVoltSignalDiag/3(GbLDP_DCPlugNegTempSTVFlt_flg) -> GbLDP_DCPlugNegTempSTVFlt_flg/1
  LowVoltSignalDiag/4(GbLDP_DCPlugNegTempSTGFlt_flg) -> GbLDP_DCPlugNegTempSTGFlt_flg/1
  LowVoltSignalDiag/5(GbLDP_CC2STG_flg) -> GbLDP_CC2STG_flg/1
  LowVoltSignalDiag/6(GbLDP_CC2VoltRaty_flg) -> GbLDP_CC2VoltRaty_flg/1
  LowVoltSignalDiag/7(GeLDP_DCPlugTempState_enum) -> GeLDP_DCPlugTempState_enum/1
  GcISP_Kl30CVolt_mV/1 -> LowVoltSignalProc/9(GcISP_Kl30CVolt_mV)
  GbISP_Kl30CVoltVld_flg/1 -> LowVoltSignalProc/10(GbISP_Kl30CVoltVld_flg)
  GbISP_HvilOutVld_flg/1 -> LowVoltSignalProc/42(GbISP_HvilOutVld_flg)
  GbISP_CshOutVld_flg/1 -> LowVoltSignalProc/46(GbISP_CshOutVld_flg)
  GbISP_HvilFbkVld_flg/1 -> LowVoltSignalProc/50(GbISP_HvilFbkVld_flg)
  GbISP_CshFbkVld_flg/1 -> LowVoltSignalProc/54(GbISP_CshFbkVld_flg)
  LowVoltSignalProc/1(GcLDP_CrntSens_mV) -> Bus Creator/1
  LowVoltSignalProc/2(GbLDP_CrntSensVld_flg) -> Bus Creator/2
  LowVoltSignalProc/3(GcLDP_HallSplyVolt_mV) -> Bus Creator/3
  LowVoltSignalProc/4(GbLDP_HallSplyVoltVld_flg) -> Bus Creator/4
  LowVoltSignalProc/5(GcLDP_CC2Volt_mV) -> Bus Creator/5
  LowVoltSignalProc/6(GbLDP_CC2VoltVld_flg) -> Bus Creator/6
  LowVoltSignalProc/7(GcLDP_DCSuplyVolt_mV) -> Bus Creator/7
  LowVoltSignalProc/8(GbLDP_DCSuplyVoltVld_flg) -> Bus Creator/8
  LowVoltSignalProc/9(GcLDP_Kl30CVolt_mV) -> Bus Creator/9
  LowVoltSignalProc/10(GbLDP_Kl30CVoltVld_flg) -> Bus Creator/10
  LowVoltSignalProc/11(GcLDP_Kl30Volt_mV) -> Bus Creator/11
  LowVoltSignalProc/12(GbLDP_Kl30VoltVld_flg) -> Bus Creator/12
  LowVoltSignalProc/13(GcLDP_PosHsdCrnt_mV) -> Bus Creator/13
  LowVoltSignalProc/14(GbLDP_PosHsdCrntVld_flg) -> Bus Creator/14
  LowVoltSignalProc/15(GcLDP_ChrgPosHsdCrnt_mV) -> Bus Creator/15
  LowVoltSignalProc/16(GbLDP_ChrgPosHsdCrntVld_flg) -> Bus Creator/16
  LowVoltSignalProc/17(GcLDP_NegHsdCrnt_mV) -> Bus Creator/17
  LowVoltSignalProc/18(GbLDP_NegHsdCrntVld_flg) -> Bus Creator/18
  LowVoltSignalProc/19(GcLDP_PosHsdVolt_mV) -> Bus Creator/19
  LowVoltSignalProc/20(GbLDP_PosHsdVoltVld_flg) -> Bus Creator/20
  LowVoltSignalProc/21(GcLDP_NegHsdVolt_mV) -> Bus Creator/21
  LowVoltSignalProc/22(GbLDP_NegHsdVoltVld_flg) -> Bus Creator/22
  LowVoltSignalProc/23(GcLDP_ChrgNegHsdCrnt_mV) -> Bus Creator/23
  LowVoltSignalProc/24(GbLDP_ChrgNegHsdCrntVld_flg) -> Bus Creator/24
  LowVoltSignalProc/25(GcLDP_ChrgPosHsdVolt_mV) -> Bus Creator/25
  LowVoltSignalProc/26(GbLDP_ChrgPosHsdVoltVld_flg) -> Bus Creator/26
  LowVoltSignalProc/27(GcLDP_ChrgNegHsdVolt_mV) -> Bus Creator/27
  LowVoltSignalProc/28(GbLDP_ChrgNegHsdVoltVld_flg) -> Bus Creator/28
  LowVoltSignalProc/29(GcLDP_BmuSplyVolt_mV) -> Bus Creator/29
  LowVoltSignalProc/30(GbLDP_BmuSplyVoltVld_flg) -> Bus Creator/30
  LowVoltSignalProc/31(GbLDP_lntWtSensVoltVld_flg) -> Bus Creator/31
  LowVoltSignalProc/32(GbLDP_OutWtSensVoltVld_flg) -> Bus Creator/32
  LowVoltSignalProc/33(GcLDP_ChrgNegTemp_mV) -> Bus Creator/33
  LowVoltSignalProc/34(GbLDP_ChrgNegTempVld_flg) -> Bus Creator/34
  LowVoltSignalProc/35(GcLDP_ChrgPosTemp_mV) -> Bus Creator/35
  LowVoltSignalProc/36(GbLDP_ChrgPosTempVld_flg) -> Bus Creator/36
  LowVoltSignalProc/37(GcLDP_HvilDutyOut_pct) -> Bus Creator/37
  LowVoltSignalProc/38(GcLDP_HvilPerOut_ms) -> Bus Creator/38
  LowVoltSignalProc/39(GcLDP_HvilSt_numb) -> Bus Creator/39
  LowVoltSignalProc/40(GcLDP_CshDutyOut_pct) -> Bus Creator/40
  LowVoltSignalProc/41(GcLDP_CshPerOut_ms) -> Bus Creator/41
  LowVoltSignalProc/42(GcLDP_CshSt_numb) -> Bus Creator/42
  LowVoltSignalProc/43(GcLDP_HvilDutyFbkt_pct) -> Bus Creator/43
  LowVoltSignalProc/44(GcLDP_HvilPerFbk_ms) -> Bus Creator/44
  LowVoltSignalProc/45(GcLDP_HvilStFbk_numb) -> Bus Creator/45
  LowVoltSignalProc/46(GcLDP_CshDutyFbk_pct) -> Bus Creator/46
  LowVoltSignalProc/47(GcLDP_CshPerFbk_ms) -> Bus Creator/47
  LowVoltSignalProc/48(GcLDP_CshStFbk_numb) -> Bus Creator/48
  LowVoltSignalProc/49(GeLDP_CC2St_enum) -> Bus Creator/49
  LowVoltSignalProc/50(GbLDP_DC12VSply_flg) -> Bus Creator/50
  LowVoltSignalProc/51(GcLDP_lntWtTemp_C) -> Bus Creator/51
  LowVoltSignalProc/52(GcLDP_OutWtTemp_C) -> Bus Creator/52
  Bus Selector/49 -> GeLDP_CC2St_enum/1  "<GeLDP_CC2St_enum>"
  Bus Selector/50 -> GbLDP_DC12VSply_flg/1  "<GbLDP_DC12VSply_flg>"
  Bus Selector/51 -> GcLDP_lntWtTemp_C/1  "<GcLDP_lntWtTemp_C>"
  Bus Selector/52 -> GcLDP_OutWtTemp_C/1  "<GcLDP_OutWtTemp_C>"
  GbISP_CrntSensL2Invld_flg/1 -> LowVoltSignalProc/55(GbISP_CrntSensL2Invld_flg)
  LowVoltSignalProc/53(GcLDP_ChrgTempNeg_C) -> Bus Creator/53
  LowVoltSignalProc/54(GcLDP_ChrgTempPos_C) -> Bus Creator/54
  Bus Selector/53 -> GcLDP_ChrgTempNeg_C/1  "<GcLDP_ChrgTempNeg_C>"
  Bus Selector/54 -> GcLDP_ChrgTempPos_C/1  "<GcLDP_ChrgTempPos_C>"
  LowVoltSignalDiag/8(GbLDP_CC2STV_flg) -> GbLDP_CC2STV_flg/1
  LowVoltSignalDiag/9(GeLDP_ChrgGunConnSt_enum) -> GeLDP_ChrgGunConnSt_enum/1
  LowVoltSignalDiag/10(GbLDP_ChrgGunConnFlt_flg) -> GbLDP_ChrgGunConnFlt_flg/1
  GeODP_ObcCcSt_enum/1 -> LowVoltSignalDiag/1(GeODP_ObcCcSt_enum)
  GbISP_TFCC2VoltRaty_flg/1 -> LowVoltSignalDiag/2(GbISP_TFCC2VoltRaty_flg)
  GbISP_TFCC2STV_flg/1 -> LowVoltSignalDiag/3(GbISP_TFCC2STV_flg)
  GbISP_TFCC2STG_flg/1 -> LowVoltSignalDiag/4(GbISP_TFCC2STG_flg)
  GeCTC_CtrCtlConnMode_enum/1 -> LowVoltSignalDiag/6(GeCTC_CtrCtlConnMode_enum)
  LowVoltSignalProc/55(LcLDP_lntWtSensVolt_mV) -> Bus Creator/55
  LowVoltSignalProc/56(LcLDP_OutWtSensVolt_mV) -> Bus Creator/56
  LowVoltSignalDiag/11(GbLDP_DCChrgPosTempSTVFlt_flg) -> GbLDP_DCChrgPosTempSTVFlt_flg/1
  LowVoltSignalDiag/12(GbLDP_DCChrgPosTempSTGFlt_flg) -> GbLDP_DCChrgPosTempSTGFlt_flg/1
  LowVoltSignalDiag/13(GbLDP_DCChrgNegTempSTVFlt_flg) -> GbLDP_DCChrgNegTempSTVFlt_flg/1
  LowVoltSignalDiag/14(GbLDP_DCChrgNegTempSTGFlt_flg) -> GbLDP_DCChrgNegTempSTGFlt_flg/1
  LowVoltSignalDiag/15(GbLDP_DCChrgPosTempHiFlt_flg) -> GbLDP_DCChrgPosTempHiFlt_flg/1
  LowVoltSignalDiag/16(GbLDP_DCChrgNegTempHiFlt_flg) -> GbLDP_DCChrgNegTempHiFlt_flg/1
  LowVoltSignalDiag/17(GbLDP_IntWtTempSTVFlt_flg) -> GbLDP_IntWtTempSTVFlt_flg/1
  LowVoltSignalDiag/18(GbLDP_IntWtTempSTGFlt_flg) -> GbLDP_IntWtTempSTGFlt_flg/1
  LowVoltSignalDiag/19(GbLDP_OutWtTempSTVFlt_flg) -> GbLDP_OutWtTempSTVFlt_flg/1
  LowVoltSignalDiag/20(GbLDP_OutWtTempSTGFlt_flg) -> GbLDP_OutWtTempSTGFlt_flg/1
  LowVoltSignalDiag/21(GbLDP_IntWtTempHiFlt_flg) -> GbLDP_IntWtTempHiFlt_flg/1
  LowVoltSignalDiag/22(GbLDP_OutWtTempHiFlt_flg) -> GbLDP_OutWtTempHiFlt_flg/1

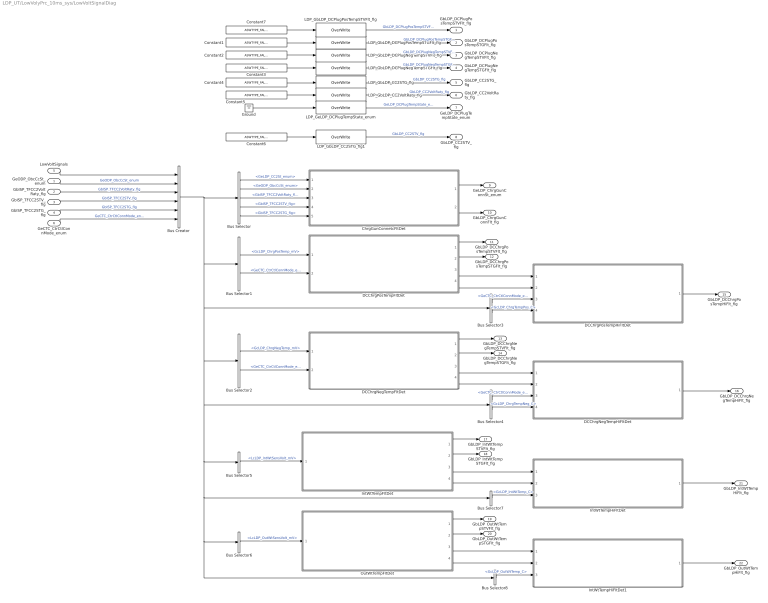
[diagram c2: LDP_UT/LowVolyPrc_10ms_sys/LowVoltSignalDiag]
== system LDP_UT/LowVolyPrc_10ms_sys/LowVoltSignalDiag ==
  GeODP_ObcCcSt_enum : Inport
  GbISP_TFCC2VoltRaty_flg : Inport  Port=2
  GbISP_TFCC2STV_flg : Inport  Port=3
  GbISP_TFCC2STG_flg : Inport  Port=4
  LowVoltSignals : Inport  Port=5
  GeCTC_CtrCtlConnMode_enum : Inport  Port=6
  Bus Creator : BusCreator  Inputs=6
  Bus Selector : BusSelector  OutputSignals=LowVoltSignals.GeLDP_CC2St_enum,GeODP_ObcCcSt_enum,GbISP_TFCC2VoltRaty_flg,GbISP_TFCC2STV_flg,GbISP_TFCC2STG_flg
  Bus Selector1 : BusSelector  OutputSignals=LowVoltSignals.GcLDP_ChrgPosTemp_mV,GeCTC_CtrCtlConnMode_enum
  Bus Selector2 : BusSelector  OutputSignals=LowVoltSignals.GcLDP_ChrgNegTemp_mV,GeCTC_CtrCtlConnMode_enum
  Bus Selector3 : BusSelector  OutputSignals=GeCTC_CtrCtlConnMode_enum,LowVoltSignals.GcLDP_ChrgTempPos_C
  Bus Selector4 : BusSelector  OutputSignals=GeCTC_CtrCtlConnMode_enum,LowVoltSignals.GcLDP_ChrgTempNeg_C
  Bus Selector5 : BusSelector  OutputSignals=LowVoltSignals.LcLDP_lntWtSensVolt_mV
  Bus Selector6 : BusSelector  OutputSignals=LowVoltSignals.LcLDP_OutWtSensVolt_mV
  Bus Selector7 : BusSelector  OutputSignals=LowVoltSignals.GcLDP_lntWtTemp_C
  Bus Selector8 : BusSelector  OutputSignals=LowVoltSignals.GcLDP_OutWtTemp_C
  ChrgGunConnetcFltDet : Subsystem
  Constant{1..7} (7 alike) : Constant  Value=ASWTYPE_FALSE
  DCChrgNegTempFltDet : Subsystem
  DCChrgNegTempHiFltDet : Subsystem
  DCChrgPosTempFltDet : Subsystem
  DCChrgPosTempHiFltDet : Subsystem
  Ground : Ground
  IntWtTempFltDet : Subsystem
  IntWtTempHiFltDet : Subsystem
  IntWtTempHiFltDet1 : Subsystem
  LDP_GbLDP_CC2STG_flg : AIWAYS_Powertrain_BMS_lib/Signals/OverWrite  OverWrite_Value=CbLDP_CC2STGOvr_flg  OverWrite_flag=CbLDP_CC2STGOvrSwt_flg
  LDP_GbLDP_CC2STG_flg1 : AIWAYS_Powertrain_BMS_lib/Signals/OverWrite  OverWrite_Value=CbLDP_CC2STVOvr_flg  OverWrite_flag=CbLDP_CC2STVOvrSwt_flg
  LDP_GbLDP_CC2VoltRaty_flg : AIWAYS_Powertrain_BMS_lib/Signals/OverWrite  OverWrite_Value=CbLDP_CC2VoltRatyOvr_flg  OverWrite_flag=CbLDP_CC2VoltRatyOvrSwt_flg
  LDP_GbLDP_DCPlugNegTempSTGFlt_flg : AIWAYS_Powertrain_BMS_lib/Signals/OverWrite  OverWrite_Value=CbLDP_DCPlugNegTempSTGFltOvr_flg  OverWrite_flag=CbLDP_DCPlugNegTempSTGFltOvrSwt_flg
  LDP_GbLDP_DCPlugNegTempSTVFlt_flg : AIWAYS_Powertrain_BMS_lib/Signals/OverWrite  OverWrite_Value=CbLDP_DCPlugNegTempSTVFltOvr_flg  OverWrite_flag=CbLDP_DCPlugNegTempSTVFltOvrSwt_flg
  LDP_GbLDP_DCPlugPosTempSTGFlt_flg : AIWAYS_Powertrain_BMS_lib/Signals/OverWrite  OverWrite_Value=CbLDP_DCPlugPosTempSTGFltOvr_flg  OverWrite_flag=CbLDP_DCPlugPosTempSTGFltOvrSwt_flg
  LDP_GbLDP_DCPlugPosTempSTVFlt_flg : AIWAYS_Powertrain_BMS_lib/Signals/OverWrite  OverWrite_Value=CbLDP_DCPlugPosTempSTVFltOvr_flg  OverWrite_flag=CbLDP_DCPlugPosTempSTVFltOvrSwt_flg
  LDP_GeLDP_DCPlugTempState_enum : AIWAYS_Powertrain_BMS_lib/Signals/OverWrite  OverWrite_Value=CeLDP_DCPlugTempStateOvr_enum  OverWrite_flag=CbLDP_DCPlugTempStateOvrSwt_flg
  OutWtTempFltDet : Subsystem
  GbLDP_DCPlugPosTempSTVFlt_flg : Outport
  GbLDP_DCPlugPosTempSTGFlt_flg : Outport  Port=2
  GbLDP_DCPlugNegTempSTVFlt_flg : Outport  Port=3
  GbLDP_DCPlugNegTempSTGFlt_flg : Outport  Port=4
  GbLDP_CC2STG_flg : Outport  Port=5
  GbLDP_CC2VoltRaty_flg : Outport  Port=6
  GeLDP_DCPlugTempState_enum : Outport  Port=7
  GbLDP_CC2STV_flg : Outport  Port=8
  GeLDP_ChrgGunConnSt_enum : Outport  Port=9
  GbLDP_ChrgGunConnFlt_flg : Outport  Port=10
  GbLDP_DCChrgPosTempSTVFlt_flg : Outport  Port=11
  GbLDP_DCChrgPosTempSTGFlt_flg : Outport  Port=12
  GbLDP_DCChrgNegTempSTVFlt_flg : Outport  Port=13
  GbLDP_DCChrgNegTempSTGFlt_flg : Outport  Port=14
  GbLDP_DCChrgPosTempHiFlt_flg : Outport  Port=15
  GbLDP_DCChrgNegTempHiFlt_flg : Outport  Port=16
  GbLDP_IntWtTempSTVFlt_flg : Outport  Port=17
  GbLDP_IntWtTempSTGFlt_flg : Outport  Port=18
  GbLDP_OutWtTempSTVFlt_flg : Outport  Port=19
  GbLDP_OutWtTempSTGFlt_flg : Outport  Port=20
  GbLDP_IntWtTempHiFlt_flg : Outport  Port=21
  GbLDP_OutWtTempHiFlt_flg : Outport  Port=22
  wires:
  Constant7/1 -> LDP_GbLDP_DCPlugPosTempSTVFlt_flg/1
  LDP_GbLDP_DCPlugPosTempSTVFlt_flg/1 -> GbLDP_DCPlugPosTempSTVFlt_flg/1  "GbLDP_DCPlugPosTempSTVFlt_flg"
  LDP_GbLDP_DCPlugNegTempSTGFlt_flg/1 -> GbLDP_DCPlugNegTempSTGFlt_flg/1  "GbLDP_DCPlugNegTempSTGFlt_flg"
  LDP_GbLDP_DCPlugNegTempSTVFlt_flg/1 -> GbLDP_DCPlugNegTempSTVFlt_flg/1  "GbLDP_DCPlugNegTempSTVFlt_flg"
  LDP_GbLDP_DCPlugPosTempSTGFlt_flg/1 -> GbLDP_DCPlugPosTempSTGFlt_flg/1  "GbLDP_DCPlugPosTempSTGFlt_flg"
  Constant3/1 -> LDP_GbLDP_DCPlugNegTempSTGFlt_flg/1
  Constant2/1 -> LDP_GbLDP_DCPlugNegTempSTVFlt_flg/1
  Constant1/1 -> LDP_GbLDP_DCPlugPosTempSTGFlt_flg/1
  LDP_GeLDP_DCPlugTempState_enum/1 -> GeLDP_DCPlugTempState_enum/1  "GeLDP_DCPlugTempState_enum"
  LDP_GbLDP_CC2VoltRaty_flg/1 -> GbLDP_CC2VoltRaty_flg/1  "GbLDP_CC2VoltRaty_flg"
  LDP_GbLDP_CC2STG_flg/1 -> GbLDP_CC2STG_flg/1  "GbLDP_CC2STG_flg"
  Constant4/1 -> LDP_GbLDP_CC2STG_flg/1
  Constant5/1 -> LDP_GbLDP_CC2VoltRaty_flg/1
  Ground/1 -> LDP_GeLDP_DCPlugTempState_enum/1
  Constant6/1 -> LDP_GbLDP_CC2STG_flg1/1
  LDP_GbLDP_CC2STG_flg1/1 -> GbLDP_CC2STV_flg/1  "GbLDP_CC2STV_flg"
  Bus Selector/1 -> ChrgGunConnetcFltDet/1(GeLDP_CC2St_enum)  "<GeLDP_CC2St_enum>"
  GeODP_ObcCcSt_enum/1 -> Bus Creator/2  "GeODP_ObcCcSt_enum"
  GbISP_TFCC2VoltRaty_flg/1 -> Bus Creator/3  "GbISP_TFCC2VoltRaty_flg"
  GbISP_TFCC2STV_flg/1 -> Bus Creator/4  "GbISP_TFCC2STV_flg"
  GbISP_TFCC2STG_flg/1 -> Bus Creator/5  "GbISP_TFCC2STG_flg"
  ChrgGunConnetcFltDet/1(GeLDP_ChrgGunConnSt_enum) -> GeLDP_ChrgGunConnSt_enum/1
  ChrgGunConnetcFltDet/2(GbLDP_ChrgGunConnFlt_flg) -> GbLDP_ChrgGunConnFlt_flg/1
  Bus Selector1/1 -> DCChrgPosTempFltDet/1(GcLDP_ChrgPosTemp_mV)  "<GcLDP_ChrgPosTemp_mV>"
  LowVoltSignals/1 -> Bus Creator/1
  GeCTC_CtrCtlConnMode_enum/1 -> Bus Creator/6  "GeCTC_CtrCtlConnMode_enum"
  Bus Selector/2 -> ChrgGunConnetcFltDet/2(GeODP_ObcCcSt_enum)  "<GeODP_ObcCcSt_enum>"
  Bus Selector/3 -> ChrgGunConnetcFltDet/3(GbISP_TFCC2VoltRaty_flg)  "<GbISP_TFCC2VoltRaty_flg>"
  Bus Selector/4 -> ChrgGunConnetcFltDet/4(GbISP_TFCC2STV_flg)  "<GbISP_TFCC2STV_flg>"
  Bus Selector/5 -> ChrgGunConnetcFltDet/5(GbISP_TFCC2STG_flg)  "<GbISP_TFCC2STG_flg>"
  Bus Selector1/2 -> DCChrgPosTempFltDet/2(GeCTC_CtrCtlConnMode_enum)  "<GeCTC_CtrCtlConnMode_enum>"
  Bus Selector2/1 -> DCChrgNegTempFltDet/1(GcLDP_ChrgNegTemp_mV)  "<GcLDP_ChrgNegTemp_mV>"
  Bus Selector2/2 -> DCChrgNegTempFltDet/2(GeCTC_CtrCtlConnMode_enum)  "<GeCTC_CtrCtlConnMode_enum>"
  DCChrgPosTempFltDet/1(GbLDP_DCChrgPosTempSTVFlt_flg) -> GbLDP_DCChrgPosTempSTVFlt_flg/1
  DCChrgPosTempFltDet/2(GbLDP_DCChrgPosTempSTGFlt_flg) -> GbLDP_DCChrgPosTempSTGFlt_flg/1
  DCChrgNegTempFltDet/1(GbLDP_DCChrgNegTempSTVFlt_flg) -> GbLDP_DCChrgNegTempSTVFlt_flg/1
  DCChrgNegTempFltDet/2(GbLDP_DCChrgNegTempSTGFlt_flg) -> GbLDP_DCChrgNegTempSTGFlt_flg/1
  Bus Selector3/1 -> DCChrgPosTempHiFltDet/3(GeCTC_CtrCtlConnMode_enum)  "<GeCTC_CtrCtlConnMode_enum>"
  DCChrgPosTempFltDet/3(LbLDP_DCChrgPosTempSTVFlt_flg) -> DCChrgPosTempHiFltDet/1(LbLDP_DCChrgPosTempSTVFlt_flg)
  DCChrgPosTempFltDet/4(LbLDP_DCChrgPosTempSTGFlt_flg) -> DCChrgPosTempHiFltDet/2(LbLDP_DCChrgPosTempSTGFlt_flg)
  Bus Selector3/2 -> DCChrgPosTempHiFltDet/4(GcLDP_ChrgTempPos_C)  "<GcLDP_ChrgTempPos_C>"
  DCChrgPosTempHiFltDet/1(GbLDP_DCChrgPosTempHiFlt_flg) -> GbLDP_DCChrgPosTempHiFlt_flg/1
  DCChrgNegTempFltDet/3(LbLDP_DCChrgNegTempSTVFlt_flg) -> DCChrgNegTempHiFltDet/1(LbLDP_DCChrgNegTempSTVFlt_flg)
  DCChrgNegTempFltDet/4(LbLDP_DCChrgNegTempSTGFlt_flg) -> DCChrgNegTempHiFltDet/2(LbLDP_DCChrgNegTempSTGFlt_flg)
  Bus Selector4/1 -> DCChrgNegTempHiFltDet/3(GeCTC_CtrCtlConnMode_enum)  "<GeCTC_CtrCtlConnMode_enum>"
  Bus Selector4/2 -> DCChrgNegTempHiFltDet/4(GcLDP_ChrgTempNeg_C)  "<GcLDP_ChrgTempNeg_C>"
  DCChrgNegTempHiFltDet/1(GbLDP_DCChrgNegTempHiFlt_flg) -> GbLDP_DCChrgNegTempHiFlt_flg/1
  Bus Selector5/1 -> IntWtTempFltDet/1(LcLDP_lntWtSensVolt_mV)  "<LcLDP_lntWtSensVolt_mV>"
  IntWtTempFltDet/1(GbLDP_IntWtTempSTVFlt_flg) -> GbLDP_IntWtTempSTVFlt_flg/1
  IntWtTempFltDet/2(GbLDP_IntWtTempSTGFlt_flg) -> GbLDP_IntWtTempSTGFlt_flg/1
  Bus Selector6/1 -> OutWtTempFltDet/1(LcLDP_OutWtSensVolt_mV)  "<LcLDP_OutWtSensVolt_mV>"
  IntWtTempFltDet/3(LbLDP_IntWtTempSTVFlt_flg) -> IntWtTempHiFltDet/1(LbLDP_IntWtTempSTVFlt_flg)
  IntWtTempFltDet/4(LbLDP_IntWtTempSTGFlt_flg) -> IntWtTempHiFltDet/2(LbLDP_IntWtTempSTGFlt_flg)
  Bus Creator/1 -> Bus Selector8/1, Bus Selector6/1, Bus Selector7/1, Bus Selector5/1, Bus Selector4/1, Bus Selector2/1, Bus Selector3/1, Bus Selector1/1, Bus Selector/1
  Bus Selector7/1 -> IntWtTempHiFltDet/3(GcLDP_lntWtTemp_C)  "<GcLDP_lntWtTemp_C>"
  OutWtTempFltDet/1(GbLDP_OutWtTempSTVFlt_flg) -> GbLDP_OutWtTempSTVFlt_flg/1
  OutWtTempFltDet/2(GbLDP_OutWtTempSTGFlt_flg) -> GbLDP_OutWtTempSTGFlt_flg/1
  IntWtTempHiFltDet/1(GbLDP_IntWtTempHiFlt_flg) -> GbLDP_IntWtTempHiFlt_flg/1
  OutWtTempFltDet/4(LbLDP_OutWtTempSTGFlt_flg) -> IntWtTempHiFltDet1/2(LbLDP_OutWtTempSTGFlt_flg)
  OutWtTempFltDet/3(LbLDP_OutWtTempSTVFlt_flg) -> IntWtTempHiFltDet1/1(LbLDP_OutWtTempSTVFlt_flg)
  Bus Selector8/1 -> IntWtTempHiFltDet1/3(GcLDP_OutWtTemp_C)  "<GcLDP_OutWtTemp_C>"
  IntWtTempHiFltDet1/1(GbLDP_OutWtTempHiFlt_flg) -> GbLDP_OutWtTempHiFlt_flg/1
